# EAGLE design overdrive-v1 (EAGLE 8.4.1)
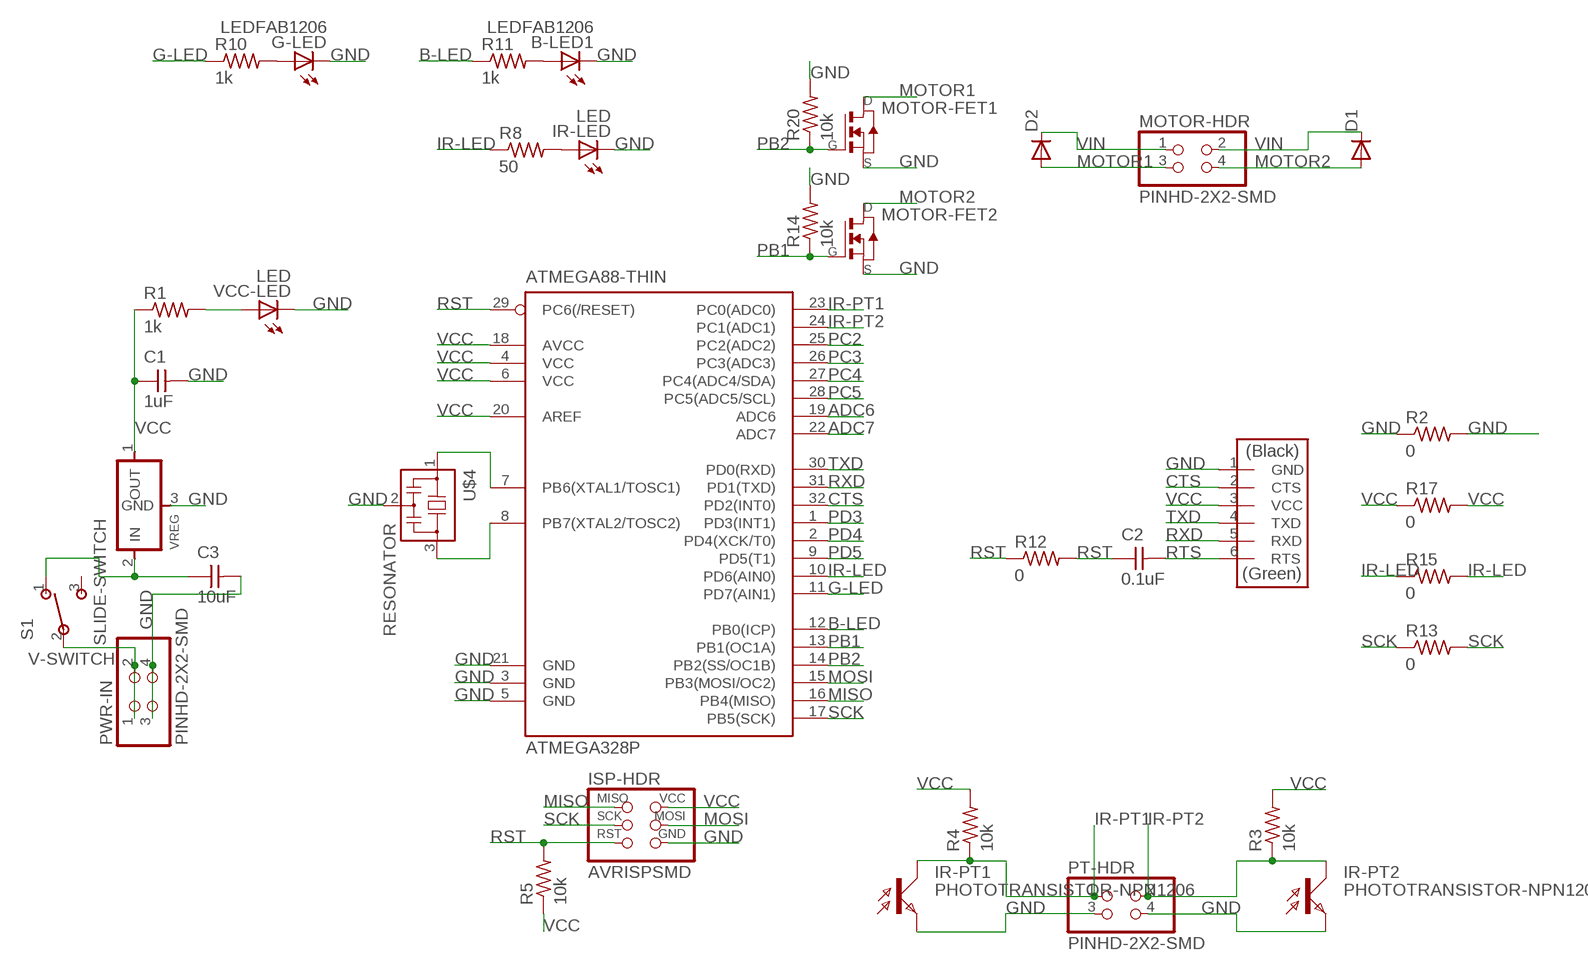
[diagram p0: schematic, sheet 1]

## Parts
ATMEGA328P  ATMEGA88-THIN  [TQFP32-08THIN]
B-LED1  LEDFAB1206  [LED1206FAB]
C1  1uF  CAP-UNPOLARIZED  [C1206]
C2  0.1uF  CAP-UNPOLARIZED  [C1206]
C3  10uF  CAP-UNPOLARIZEDFAB  [C1206FAB]
D1  DIODESOD123  [SOD123]
D2  DIODESOD123  [SOD123]
G-LED  LEDFAB1206  [LED1206FAB]
IR-LED  LED  [LED1206]
IR-PT1  PHOTOTRANSISTOR-NPN1206  [OP1206]
IR-PT2  PHOTOTRANSISTOR-NPN1206  [OP1206]
ISP-HDR  AVRISPSMD  [2X03SMD]
MOTOR-FET1  NMOSFETSOT23  [SOT-23]
MOTOR-FET2  NMOSFETSOT23  [SOT-23]
MOTOR-HDR  PINHD-2X2-SMD  [2X02SMD]
PT-HDR  PINHD-2X2-SMD  [2X02SMD]
PWR-IN  PINHD-2X2-SMD  [2X02SMD]
R1  1k  RES-US1206FAB  [R1206FAB]
R2  0  RES-US1206FAB  [R1206FAB]
R3  10k  RES-US1206FAB  [R1206FAB]
R4  10k  RES-US1206FAB  [R1206FAB]
R5  10k  RES-US1206FAB  [R1206FAB]
R8  50  RES-US1206FAB  [R1206FAB]
R10  1k  RES-US1206FAB  [R1206FAB]
R11  1k  RES-US1206FAB  [R1206FAB]
R12  0  RES-US1206FAB  [R1206FAB]
R13  0  RES-US1206FAB  [R1206FAB]
R14  10k  RES-US1206FAB  [R1206FAB]
R15  0  RES-US1206FAB  [R1206FAB]
R17  0  RES-US1206FAB  [R1206FAB]
R20  10k  RES-US1206FAB  [R1206FAB]
S1  SLIDE-SWITCH  [AYZ0102AGRLC]
U$4  RESONATOR  [EFOBM]
U$6  FTDI-SMD-HEADER  [1X06SMD]
VCC-LED  LED  [LED1206]
VREG  REGULATORSOT23  [SOT23]

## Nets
ADC6: ATMEGA328P.19(ADC6)
ADC7: ATMEGA328P.22(ADC7)
B-LED: ATMEGA328P.12(PB0(ICP)) R11.1
CTS: ATMEGA328P.32(PD2(INT0)) U$6.2(CTS)
G-LED: ATMEGA328P.11(PD7(AIN1)) R10.1
GND: ATMEGA328P.3(GND) ATMEGA328P.5(GND) ATMEGA328P.21(GND) B-LED1.2(C) C1.2 C3.2 G-LED.2(C) IR-LED.2(C) IR-PT1.EMITTER(E) IR-PT2.EMITTER(E) ISP-HDR.6(GND) MOTOR-FET1.2(S) MOTOR-FET2.2(S) PT-HDR.3 PT-HDR.4 PWR-IN.3 PWR-IN.4 R2.1 R2.2 R14.2 R20.2 U$4.2 U$6.1(GND) VCC-LED.2(C) VREG.3(GND)
IR-LED: ATMEGA328P.10(PD6(AIN0)) R8.1 R15.1 R15.2
IR-PT1: ATMEGA328P.23(PC0(ADC0)) IR-PT1.COLLECTOR(C) PT-HDR.1 R4.1
IR-PT2: ATMEGA328P.24(PC1(ADC1)) IR-PT2.COLLECTOR(C) PT-HDR.2 R3.1
MISO: ATMEGA328P.16(PB4(MISO)) ISP-HDR.1(MISO)
MOSI: ATMEGA328P.15(PB3(MOSI/OC2)) ISP-HDR.4(MOSI)
MOTOR1: D2.ANODE(A) MOTOR-FET1.1(D) MOTOR-HDR.3
MOTOR2: D1.ANODE(A) MOTOR-FET2.1(D) MOTOR-HDR.4
N$1: R1.2 VCC-LED.1(A)
N$2: ATMEGA328P.7(PB6(XTAL1/TOSC1)) U$4.1
N$3: ATMEGA328P.8(PB7(XTAL2/TOSC2)) U$4.3
N$9: IR-LED.1(A) R8.2
N$11: G-LED.1(A) R10.2
N$13: B-LED1.1(A) R11.2
PB1: ATMEGA328P.13(PB1(OC1A)) MOTOR-FET2.3(G) R14.1
PB2: ATMEGA328P.14(PB2(SS/OC1B)) MOTOR-FET1.3(G) R20.1
PC2: ATMEGA328P.25(PC2(ADC2))
PC3: ATMEGA328P.26(PC3(ADC3))
PC4: ATMEGA328P.27(PC4(ADC4/SDA))
PC5: ATMEGA328P.28(PC5(ADC5/SCL))
PD3: ATMEGA328P.1(PD3(INT1))
PD4: ATMEGA328P.2(PD4(XCK/T0))
PD5: ATMEGA328P.9(PD5(T1))
RST: ATMEGA328P.29(PC6(/RESET)) C2.1 ISP-HDR.5(RST) R5.2 R12.1 R12.2
RTS: C2.2 U$6.6(RTS)
RXD: ATMEGA328P.31(PD1(TXD)) U$6.5(RXD)
SCK: ATMEGA328P.17(PB5(SCK)) ISP-HDR.3(SCK) R13.1 R13.2
TXD: ATMEGA328P.30(PD0(RXD)) U$6.4(TXD)
V-SWITCH: PWR-IN.1 PWR-IN.2 S1.2
VCC: ATMEGA328P.4(VCC) ATMEGA328P.6(VCC) ATMEGA328P.18(AVCC) ATMEGA328P.20(AREF) C1.1 ISP-HDR.2(VCC) R1.1 R3.2 R4.2 R5.1 R17.1 R17.2 U$6.3(VCC) VREG.1(OUT)
VIN: C3.1 D1.CATHODE(C) D2.CATHODE(C) MOTOR-HDR.1 MOTOR-HDR.2 S1.1 VREG.2(IN)
Unconnected: S1.3

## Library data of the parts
ATMEGA328P = fab:ATMEGA88-THIN
B-LED1 G-LED IR-LED VCC-LED = fab:LED: LED
C1-C3 = fab:CAP-UNPOLARIZED
D1 D2 = fab:DIODE: DIODE
IR-PT1 IR-PT2 = fab:PHOTOTRANSISTOR-NPN
ISP-HDR = fab:AVRISP
MOTOR-FET1 MOTOR-FET2 = fab:NMOSFET: MOS FET
MOTOR-HDR PT-HDR PWR-IN = fab:PINHD-2X2-SMD
R1-R5 R8 R10-R15 R17 R20 = fab:RES-US: Resistor (US Symbol)
S1 = fab:SLIDE-SWITCH: SMD slide-switch AYZ0102AGRLC as found in the fablab inventory. Includes the mounting holes. Made by Zaerc.
U$4 = fab:RESONATOR
U$6 = fab:FTDI-SMD-HEADER
VREG = fab:REGULATOR

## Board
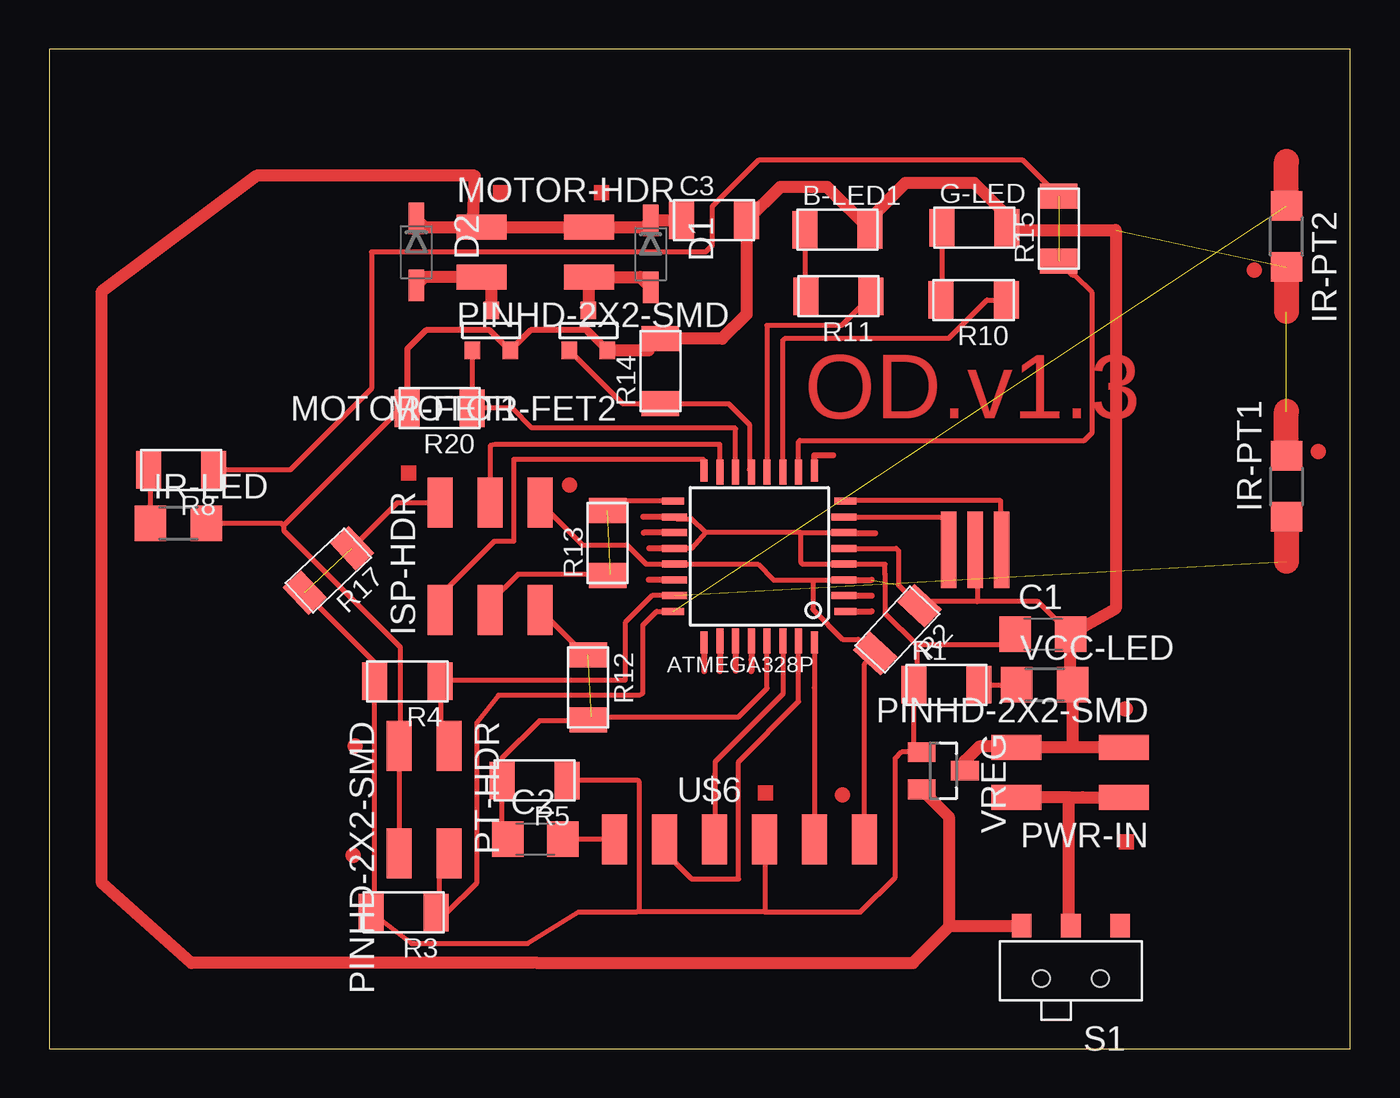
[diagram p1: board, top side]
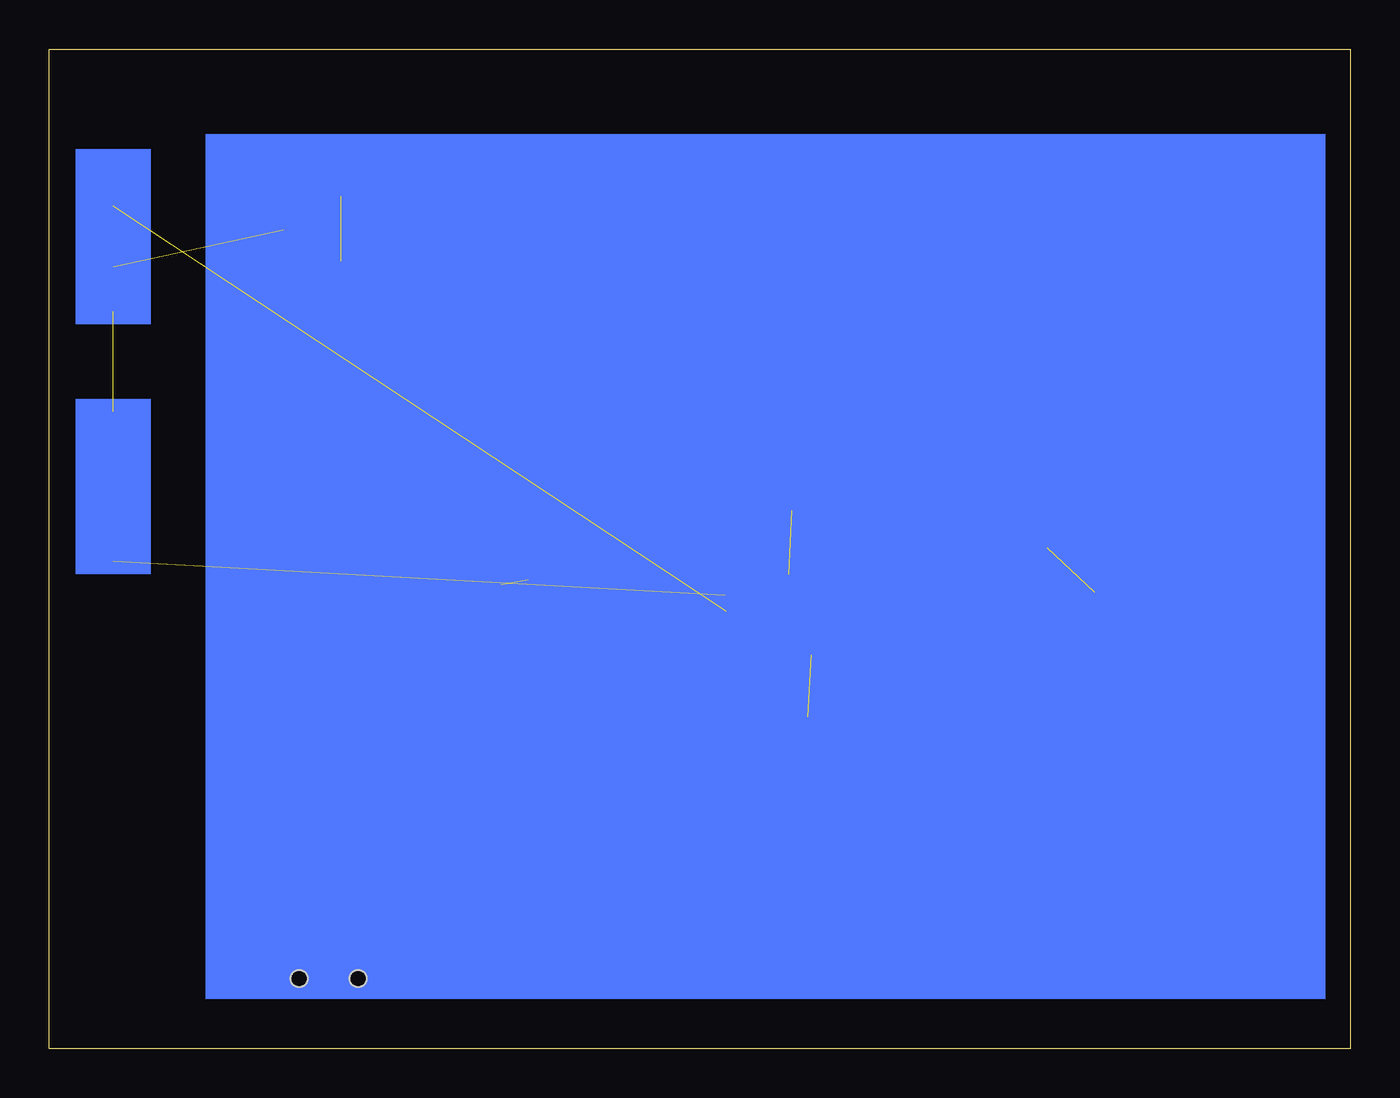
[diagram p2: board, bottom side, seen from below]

Size 66.11 x 50.79 mm. Coordinates in mm from the lower left corner, seen from the top.
Outline: 0,0 66.11,0 66.11,50.79 0,50.79 0,0
Copper layers (1*16): Top 0.035mm / dielectric 1.5mm / Bottom 0.035mm
Design rules "default *": minimum track width 10mil, minimum drill 0.35mm, track to track 0.397003125mm, track to pad 0.397003125mm, pad to pad 0.397003125mm, via to via 0.397003125mm, smd to smd 6mil, copper to edge 15.625mil, drill to drill 15.625mil, minimum pad ring 10mil, minimum via ring 8mil, stop-mask expansion 4mil, vias tented up to drill 0mil, thermal gap 10mil

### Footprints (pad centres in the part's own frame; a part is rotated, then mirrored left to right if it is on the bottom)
TQFP32-08THIN = smd 1.118 x 0.356: 1 -4.369,2.8; 8 -4.369,-2.8; 17 4.369,-2.8; 24 4.369,2.8 | smd 1.27 x 0.356: 2 -4.293,2; 3 -4.293,1.2; 4 -4.293,0.4; 5 -4.293,-0.4; 6 -4.293,-1.2; 7 -4.293,-2; 18 4.293,-2; 19 4.293,-1.2; 20 4.293,-0.4; 21 4.293,0.4; 22 4.293,1.2; 23 4.293,2 | smd 0.356 x 1.118: 9 -2.8,-4.369; 16 2.8,-4.369; 25 2.8,4.369; 32 -2.8,4.369 | smd 0.356 x 1.27: 10 -2,-4.293; 14 1.2,-4.293; 15 2,-4.293; 26 2,4.293; 27 1.2,4.293; 31 -2,4.293 | smd 0.35 x 1.27: 11 -1.2,-4.293; 12 -0.4,-4.293; 13 0.4,-4.293; 28 0.4,4.293; 29 -0.4,4.293; 30 -1.2,4.293
LED1206FAB = smd 1.27 x 1.905: 1 -1.651,0; 2 1.651,0
C1206 = smd 1.6 x 1.8: 1 -1.4,0; 2 1.4,0
C1206FAB = smd 1.27 x 1.905: 1 -1.651,0; 2 1.651,0
SOD123 = smd 1.6 x 0.8: ANODE 1.7,0; CATHODE -1.7,0
LED1206 = smd 1.6 x 1.803: 1 -1.422,0; 2 1.422,0
OP1206 = smd 1.5 x 1.6: COLLECTOR -1.55,0; EMITTER 1.55,0
2X03SMD = smd 2.54 x 1.27: 1 -2.54,2.54; 2 2.92,2.54; 3 -2.54,0; 4 2.92,0; 5 -2.54,-2.54; 6 2.92,-2.54
SOT-23 = smd 0.787 x 0.889: 1 0.025,-1.016; 2 -0.94,1.016; 3 0.991,1.016
2X02SMD = smd 2.54 x 1.27: 1 -2.54,1.27; 2 2.92,1.27; 3 -2.54,-1.27; 4 2.92,-1.27
R1206FAB = smd 1.27 x 1.905: 1 -1.651,0; 2 1.651,0
AYZ0102AGRLC = smd 1 x 1.2: 1 2.5,-2.3; 2 0,-2.3; 3 -2.5,-2.3 | hole 0.85: -1.5,0.4; 1.5,0.4
EFOBM = smd 0.8 x 3.9: 1 -1.35,0; 2 0,0; 3 1.35,0
1X06SMD = smd 2.54 x 1.27: 1 0,6.35; 2 0,3.81; 3 0,1.27; 4 0,-1.27; 5 0,-3.81; 6 0,-6.35
SOT23 = smd 1 x 1.4: 1 -0.95,-1.1; 2 0.95,-1.1; 3 0,1.1

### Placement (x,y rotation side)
ATMEGA328P  36.08,25.02 180 top
B-LED1  40.04,41.61 0 top
C1  50.49,21.07 0 top
C2  24.71,10.66 0 top
C3  33.78,42.1 0 top
D1  30.56,40.38 270 top
D2  18.65,40.48 270 top
G-LED  47.01,41.71 0 top
IR-LED  6.57,26.69 0 top
IR-PT1  62.87,28.57 90 top
IR-PT2  62.87,41.27 270 top
ISP-HDR  22.4,24.82 90 top
MOTOR-FET1  22.48,36.49 180 top
MOTOR-FET2  27.42,36.49 180 top
MOTOR-HDR  24.51,40.48 0 top
PT-HDR  19.05,12.84 270 top
PWR-IN  52.06,14.05 180 top
R1  45.58,18.49 0 top
R2  43.09,21.3 227.1 top
R3  18,6.92 180 top
R4  18.2,18.67 180 top
R5  24.67,13.63 180 top
R8  6.71,29.41 180 top
R10  46.97,38.04 180 top
R11  40.1,38.24 180 top
R12  27.38,18.36 270 top
R13  28.38,25.7 90 top
R14  31.06,34.43 90 top
R15  51.3,41.67 90 top
R17  14.19,24.31 223.2 top
R20  19.84,32.54 180 top
S1  51.91,3.96 180 top
U$4  47.05,25.36 0 top
U$6  35.08,10.64 270 top
VCC-LED  50.59,18.49 0 top
VREG  45.42,14.12 270 top

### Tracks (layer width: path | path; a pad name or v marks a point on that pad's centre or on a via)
ADC6
  Top 0.305: ATMEGA328P.19 30.21,26.22
ADC7
  Top 0.305: ATMEGA328P.22 30.47,23.82
B-LED
  Top 0.254: 41.41,38.24 R11.1 40.26,36.75 36.45,36.75 36.48,36.73 ATMEGA328P.12
CTS
  Top 0.254: ATMEGA328P.32 38.88,18.34 38.89,18.32 U$6.2
G-LED
  Top 0.254: ATMEGA328P.11 37.28,35.99 37.39,36.1 45.71,36.1 47.65,38.04 R10.1
GND  (3 unrouted)
  Top 0.254: 38.8,23.81 36.81,23.81 36,24.62 ATMEGA328P.21 30.33,24.62 29.35,25.6 27.09,25.6 ISP-HDR.6 | 38.8,23.81 40.36,23.81 ATMEGA328P.3 | ATMEGA328P.5 43.04,25.42 43.16,25.3 43.16,23.56 R2.1 44.43,22.72 47.15,22.72 | 17.78,15.26 17.78,15.35 | 17.78,15.26 PT-HDR.4 | 17.78,15.35 PT-HDR.3 17.78,15.8 | 41.47,10.68 U$6.1 | 38.8,23.81 38.8,22.32 40.32,20.8 41.11,20.8 41.82,20.09 R2.2 41.43,19.55 U$6.1 | R14.2 30.45,35.48 | 27.38,36.46 27.38,36.51 | 17.65,32.54 R20.2 17.88,32.54 11.91,26.58 | 34.2,36.08 34.23,36.12 | 11.91,26.58 11.8,26.69 IR-LED.2 | U$6.1 41.51,10.56 | C1.2 50.24,22.72 47.15,22.72 | 18.23,15.8 17.78,15.35 | 11.91,26.58 11.91,26.32 17.83,20.41 17.83,15.31 17.78,15.26 | U$4.2 47.15,25.25 47.15,22.72
  Top 0.305: 27.38,36.51 24.46,36.51 MOTOR-FET1.2 22.39,36.51 19.15,36.51 18.19,35.56 R20.2 | ATMEGA328P.3 41.79,23.82
  Top 0.406: 23.47,35.48 MOTOR-FET1.2 | 31.12,36.08 R14.2 | MOTOR-FET2.2 27.38,36.46
  Top 0.61: PWR-IN.3 52.11,15.32 | 52.11,15.32 PWR-IN.4 49.1,15.35 47.25,15.35 46.52,14.63 VREG.3 | 41.75,41.67 B-LED1.2 | 30.45,35.48 MOTOR-FET2.2 | R14.2 34.2,36.08 35.43,37.32 C3.2 35.46,42.1 37.15,43.78 39.52,43.78 B-LED1.2 | B-LED1.2 41.69,42.19 43.49,43.98 47,43.98 48.66,42.32 G-LED.2 48.77,41.6 54.19,41.6 54.19,22.38 C1.2 | 52.11,15.32 52.01,15.41 VCC-LED.2 51.89,18.61 C1.2 | C1.2 51.81,21.15
  Top 1.27: IR-PT2.EMITTER 62.87,37.47 | IR-PT1.EMITTER 62.87,32.38
IR-LED  (1 unrouted)
  Top 0.254: R15.2 49.47,45.15 36.03,45.15 33.68,42.79 33.68,40.81 33.35,40.48 16.37,40.48 16.37,33.54 12.24,29.41 R8.1 | ATMEGA328P.10 38.08,30.84 38.14,30.91 52.6,30.91 53,31.3 53,38.42 52.12,39.3 52.02,39.3 R15.1
IR-PT1  (1 unrouted)
  Top 0.254: ATMEGA328P.23 31.68,23.02 30.64,23.02 29.27,21.66 29.27,18.75 29.24,18.72 19.9,18.72 | 19.9,18.72 R4.1 | PT-HDR.1 19.9,15.8 19.9,18.72
  Top 1.27: IR-PT1.COLLECTOR 62.87,24.77
IR-PT2  (1 unrouted)
  Top 0.254: ATMEGA328P.24 30.86,22.22 30.16,21.53 30.16,18.06 29.97,17.96 26.21,17.96 22.82,17.96 21.73,16.57 21.73,8.43 20.22,6.92 19.81,6.92 | 19.81,6.92 R3.1 | PT-HDR.2 19.81,9.41 19.81,6.92
  Top 1.27: IR-PT2.COLLECTOR 62.87,45.09
MISO
  Top 0.254: ISP-HDR.1 19.86,23.04 22.62,25.8 23.61,25.8 23.61,29.96 23.9,29.95 33.24,29.95 33.24,29.43 ATMEGA328P.16
MOSI
  Top 0.254: ATMEGA328P.15 34.08,30.7 22.66,30.7 22.4,30.64 ISP-HDR.4
MOTOR1
  Top 0.61: MOTOR-FET1.1 22.46,39.4 MOTOR-HDR.3 19.08,39.21 D2.ANODE
MOTOR2
  Top 0.61: 27.4,39.18 MOTOR-FET2.1 | 27.4,39.18 MOTOR-HDR.4 30.03,39.21 D1.ANODE | 27.6,38.98 27.4,39.18
N$1
  Top 0.254: R1.2 VCC-LED.1
N$2
  Top 0.254: 40.43,27.09 ATMEGA328P.7 45.74,27.02 45.77,27.04 45.7,26.98 U$4.1
N$3
  Top 0.254: ATMEGA328P.8 40.5,27.88 48.3,27.88 48.34,27.84 48.34,25.42 U$4.3
N$9
  Top 0.254: 5.04,29.43 R8.2 5.15,29.32 IR-LED.1
N$11
  Top 0.254: G-LED.1 45.36,38.08 R10.2
N$13
  Top 0.254: B-LED1.1 38.39,38.3 R11.2
PB1
  Top 0.254: ATMEGA328P.13 35.58,29.41 35.58,31.72 35.53,31.77 | MOTOR-FET2.3 29.13,32.78 R14.1 34.52,32.78 35.09,32.2 | 35.09,32.2 | 35.53,31.77 | 35.09,32.2 35.53,31.77
PB2
  Top 0.254: ATMEGA328P.14 34.88,31.5 34.83,31.55 24.52,31.55 23.53,32.54 R20.1 MOTOR-FET1.3
PC2
  Top 0.305: ATMEGA328P.25 33.28,19.19
PC3
  Top 0.305: ATMEGA328P.26 34.08,19.19
PC4
  Top 0.305: ATMEGA328P.27 34.88,19.2
PC5
  Top 0.305: ATMEGA328P.28 35.68,19.77 35.68,19.19
PD3
  Top 0.305: ATMEGA328P.1 | ATMEGA328P.1 41.79,22.23
PD4
  Top 0.305: ATMEGA328P.2 41.79,23.02
PD5
  Top 0.305: ATMEGA328P.9 38.88,30.16 39.82,30.16
RST  (1 unrouted)
  Top 0.254: 23.02,13.49 R5.2 23.02,14.78 24.9,16.67 27.35,16.67 R12.2 27.55,16.87 35.02,16.87 36.48,18.32 ATMEGA328P.29 | 23.16,13.64 23.02,13.49 | 27.32,20.07 R12.1 27.22,20.01 ISP-HDR.5 | C2.1 23.02,10.95 23.02,13.49
RTS
  Top 0.254: C2.2 28.71,10.66 U$6.6
RXD
  Top 0.254: ATMEGA328P.31 38.08,17.64 35.02,14.59 35.02,8.63 32.64,8.63 31.27,10 U$6.5
SCK  (1 unrouted)
  Top 0.254: ATMEGA328P.17 29.25,27.82 R13.2 | R13.1 28.51,24.11 23.81,24.11 22.4,22.7 ISP-HDR.3
TXD
  Top 0.254: 33.83,13.89 33.83,13.99 | 33.83,13.89 33.83,10.66 U$6.4 | 33.83,13.89 33.83,14.59 37.28,18.03 ATMEGA328P.30
V-SWITCH
  Top 0.61: 52.5,12.78 PWR-IN.1 | 51.81,12.78 52.5,12.78 | 51.81,12.78 PWR-IN.2 | 52.5,12.78 | S1.2 51.81,6.36 51.81,12.78
VCC  (1 unrouted)
  Top 0.254: ATMEGA328P.20 31.88,25.42 32.63,25.42 33.34,26.22 | 38.2,26.22 ATMEGA328P.6 40.4,26.19 | 38.2,26.22 33.34,26.22 | ATMEGA328P.18 31.88,26.93 32.63,26.93 33.34,26.22 | 38.2,26.22 38.2,24.7 38.28,24.62 ATMEGA328P.4 42.45,24.62 | 42.45,24.62 42.47,24.61 | R5.1 29.92,13.63 29.96,13.59 29.96,7.04 29.86,6.95 | R17.1 17.7,27.75 ISP-HDR.2 | 29.86,6.95 26.89,6.95 24.31,5.36 18.41,5.36 R3.2 16.55,7.12 R4.2 | R4.2 16.44,18.78 | 12.98,23.07 R17.2 16.55,19.62 R4.2 | 42.45,24.62 42.45,24.12 42.47,24.1 42.47,22.12 44.08,20.5 | 44.08,20.5 44.08,18.64 R1.1 43.93,15.47 VREG.1 43.31,15.07 42.99,14.76 42.99,8.72 41.22,6.95 36.35,6.95 | C1.1 48.52,20.5 44.08,20.5 | 36.35,6.95 29.86,6.95 | U$6.3 36.35,6.95
  Top 0.305: 40.4,26.19 41.97,26.19 | ATMEGA328P.18 30.18,27.02 | ATMEGA328P.20 30.48,25.42
VIN
  Top 0.61: D2.CATHODE 19.08,41.75 MOTOR-HDR.1 | MOTOR-HDR.1 MOTOR-HDR.2 30.23,41.75 D1.CATHODE 32.11,42.08 C3.1 | MOTOR-HDR.1 21.53,42.19 21.63,44.35 10.52,44.35 2.67,38.49 2.67,8.42 7.23,4.36 24.8,4.36 25.6,4.37 43.89,4.37 45.77,6.24 | S1.1 49.39,6.24 45.77,6.24 | 45.77,6.24 45.71,6.24 45.71,11.79 VREG.2
(copper drawn outside any net)
  shapes: Bottom area x3, Top area x5, Top circle x7

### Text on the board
Top: OD.v1.3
